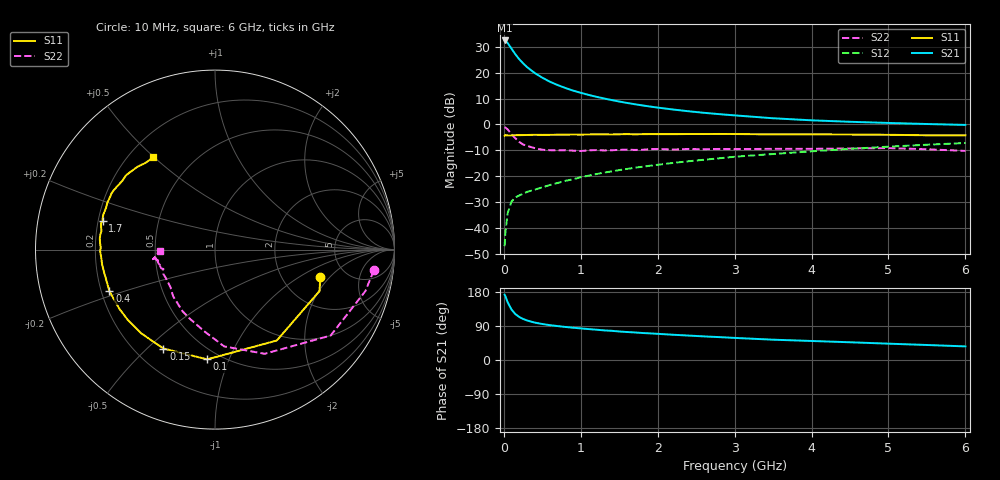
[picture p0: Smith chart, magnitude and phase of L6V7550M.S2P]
!  INFINEON TECHNOLOGIES Small Signal Semiconductors
! BFR380L3 , Si-NPN RF-Transistor in TSLP-3-1
!  Vce=0.75 V,  Ic=50 mA
! Common Emitter S-Parameters:  07. March 2005
#  GHz  S  MA  R  50
! f  S11  S21  S12  S22
! GHz  Mag  Ang  Mag  Ang  Mag  Ang  Mag  Ang
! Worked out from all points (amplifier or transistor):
!   36 points, 10 MHz to 6 GHz, reference 50 ohm
!   highest |S21| = 32.4 dB at 10 MHz (marker M1)
!   |S21| within 3 dB of that: start of sweep to 96.11 MHz
!   unconditionally stable (mu >= 1): 1.074 GHz to end of sweep
!   at 250 MHz: K = 0.53, MSG = 25.2 dB, |S12| = -26.7 dB
!   at 1.4 GHz: K = 1.04, MAG = 12.5 dB, |S12| = -18.1 dB
!   at 6 GHz: K = 1.01, MAG = 2.8 dB, |S12| = -7.1 dB
!   S11 on the Smith chart (normalised r, x): 10 MHz: 3.24, -1.59; 100 MHz: 0.43, -0.84; 150 MHz: 0.31, -0.56; 400 MHz: 0.23, -0.18; 1.7 GHz: 0.22, +0.12; 6 GHz: 0.30, +0.50
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0.01  0.6065 -14.8  41.67 172.3  0.0045 76.9  0.8921 -7.5
0.02  0.6265 -21.6  41.14 168.4  0.0083 78.3  0.8694 -15.4
0.05  0.6126 -55.8  37.08 152.2  0.0195 67.8  0.8028 -36.6
0.1  0.6131 -94.1  28.94 133.1  0.0328 53.9  0.6432 -64.5
0.15  0.6214 -117.5  22.56 121.1  0.0394 48.1  0.5416 -84.6
0.2  0.6219 -131.3  18.14 113.6  0.0428 46.1  0.4612 -97.0
0.25  0.6242 -141.3  15.11 108.4  0.0461 44.8  0.4111 -109.6
0.3  0.6266 -148.3  12.81 104.4  0.0501 46.5  0.3885 -117.6
0.4  0.6323 -158.4  9.852 98.8  0.0552 48.3  0.3497 -131.8
0.5  0.6293 -164.7  7.977 95.0  0.0614 51.0  0.3255 -139.4
0.6  0.6313 -169.3  6.651 91.9  0.0681 52.8  0.3189 -145.3
0.7  0.6342 -172.6  5.747 89.5  0.0745 55.3  0.3165 -150.8
0.9  0.6401 -179.2  4.491 85.2  0.0877 58.5  0.3132 -158.2
1.1  0.6416 176.6  3.719 81.6  0.1029 60.5  0.3174 -160.9
1.4  0.6413 170.8  2.959 77.1  0.1241 62.1  0.3179 -165.0
1.7  0.6455 165.7  2.46 72.7  0.1464 63.0  0.3232 -169.4
2.2  0.6499 159.0  1.942 66.6  0.1813 63.1  0.3282 -169.8
2.8  0.6561 151.5  1.581 60.4  0.2226 62.8  0.3373 -172.6
3.5  0.6431 143.4  1.317 53.6  0.2692 60.3  0.3388 -172.0
4.5  0.6389 137.0  1.126 46.8  0.3388 57.7  0.3447 -171.7
5.5  0.6187 128.6  1.02 39.6  0.4066 53.0  0.3327 -173.5
6  0.6193 123.6  0.98 35.9  0.4394 50.5  0.3089 -178.5
